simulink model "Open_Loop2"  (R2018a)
settings: Solver=VariableStepAuto  StartTime=0.0  StopTime=50  FixedStep=Ts  MaxStep=0.05  RelTol=1e-3  EnableMultiTasking=on
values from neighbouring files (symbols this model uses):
  Ax = 54.8    [init.m]
  Mlh2 = 41.12    [init.m]
  Mlox = 119.3    [init.m]
  Zeta = 0.002    [init.m]
undefined symbols (not defined in the file or in its folder): Aa, Av2, Ba, Bv2, Ca, Cv2, Da, Dv2, Kmix, Kq

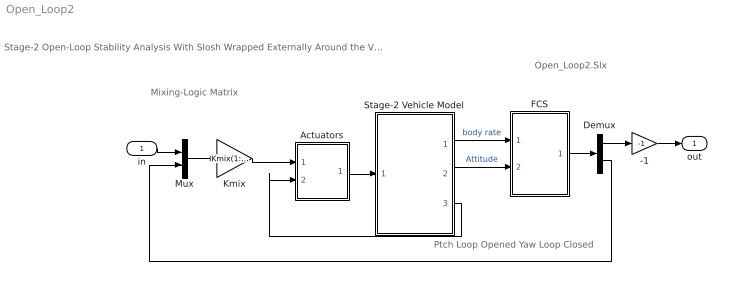
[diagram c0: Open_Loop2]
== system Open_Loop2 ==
  note: Stage-2 Open-Loop Stability Analysis With Slosh Wrapped Externally Around the Vehicle
  note: Mixing-Logic Matrix
  note: Ptch Loop Opened Yaw Loop Closed
  note: Open_Loop2.Slx
  in : Inport
  -1 : Gain  Gain=-1
  Actuators : Subsystem
  Demux : Demux  Outputs=2
  FCS : Subsystem
  Kmix : Gain  Gain=Kmix(1:2,2:3)  Multiplication=Matrix(K*u)
  Mux : Mux  Inputs=2
  Stage-2 Vehicle Model : Subsystem
  out : Outport
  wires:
  Stage-2 Vehicle Model/1(Wb) -> FCS/1(rate)  "body rate"
  Stage-2 Vehicle Model/2(atti) -> FCS/2(atter)  "Attitude"
  FCS/1(DQ,DR) -> Demux/1
  -1/1 -> out/1
  Actuators/1(del) -> Stage-2 Vehicle Model/1(dy,dz)
  Kmix/1 -> Actuators/1(dc)
  Mux/1 -> Kmix/1
  in/1 -> Mux/1
  Demux/1 -> -1/1
  Demux/2 -> Mux/2
  Stage-2 Vehicle Model/3(TL) -> Actuators/2(TL)

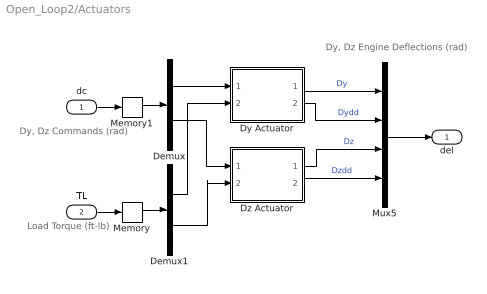
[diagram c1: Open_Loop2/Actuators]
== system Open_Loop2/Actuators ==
  note: Dy, Dz Engine Deflections (rad)
  note: Load Torque (ft-lb)
  note: Dy, Dz Commands (rad)
  dc : Inport
  TL : Inport  Port=2
  Demux : Demux  Outputs=2
  Demux1 : Demux  Outputs=2
  Dy Actuator : Subsystem
  Dz Actuator : Subsystem
  Memory : Memory
  Memory1 : Memory
  Mux5 : Mux
  del : Outport
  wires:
  Demux1/1 -> Dy Actuator/2(TL)
  Mux5/1 -> del/1
  Demux1/2 -> Dz Actuator/2(TL)
  Demux/2 -> Dz Actuator/1(dc)
  Dy Actuator/1(del) -> Mux5/1  "Dy"
  Dy Actuator/2(ddd) -> Mux5/2  "Dydd"
  Demux/1 -> Dy Actuator/1(dc)
  Dz Actuator/1(del) -> Mux5/3  "Dz"
  Dz Actuator/2(ddd) -> Mux5/4  "Dzdd"
  dc/1 -> Memory1/1
  TL/1 -> Memory/1
  Memory/1 -> Demux1/1
  Memory1/1 -> Demux/1

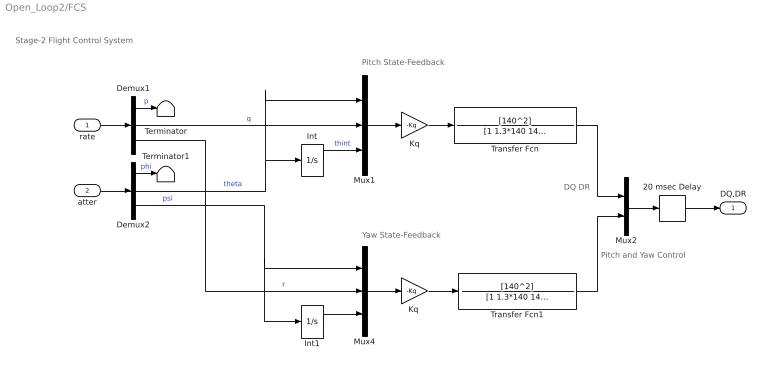
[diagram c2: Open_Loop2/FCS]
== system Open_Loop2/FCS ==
  note: Stage-2 Flight Control System
  note: Pitch and Yaw Control
  note: Yaw State-Feedback
  note: Pitch State-Feedback
  note: DQ DR
  rate : Inport
  atter : Inport  Port=2
  20 msec Delay : TransportDelay  DelayTime="[1  1]*0.020"  InitialOutput=[0 0]  PadeOrder=2
  Demux1 : Demux  Outputs=3
  Demux2 : Demux  Outputs=3
  Int : Integrator
  Int1 : Integrator
  Kq : Gain  Gain=-Kq  Multiplication=Matrix(K*u)
  "Kq " : Gain  Gain=-Kq  Multiplication=Matrix(K*u)
  Mux1 : Mux  Inputs=3
  Mux2 : Mux  Inputs=2
  Mux4 : Mux  Inputs=3
  Terminator : Terminator
  Terminator1 : Terminator
  Transfer Fcn : TransferFcn  Numerator=[140^2]  Denominator=[1 1.3*140 140^2]
  Transfer Fcn1 : TransferFcn  Numerator=[140^2]  Denominator=[1 1.3*140 140^2]
  DQ,DR : Outport
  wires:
  20 msec Delay/1 -> DQ,DR/1
  Demux2/1 -> Terminator1/1  "phi"
  Demux1/1 -> Terminator/1  "p"
  "Kq "/1 -> Transfer Fcn1/1
  Mux4/1 -> "Kq "/1
  Transfer Fcn1/1 -> Mux2/2
  Transfer Fcn/1 -> Mux2/1
  Mux1/1 -> Kq/1
  atter/1 -> Demux2/1
  Demux2/3 -> Mux4/1, Int1/1  "psi"
  Demux1/3 -> Mux4/2  "r"
  Int1/1 -> Mux4/3
  Int/1 -> Mux1/3  "thint"
  Demux1/2 -> Mux1/2  "q"
  Demux2/2 -> Int/1, Mux1/1  "theta"
  Kq/1 -> Transfer Fcn/1
  rate/1 -> Demux1/1
  Mux2/1 -> 20 msec Delay/1

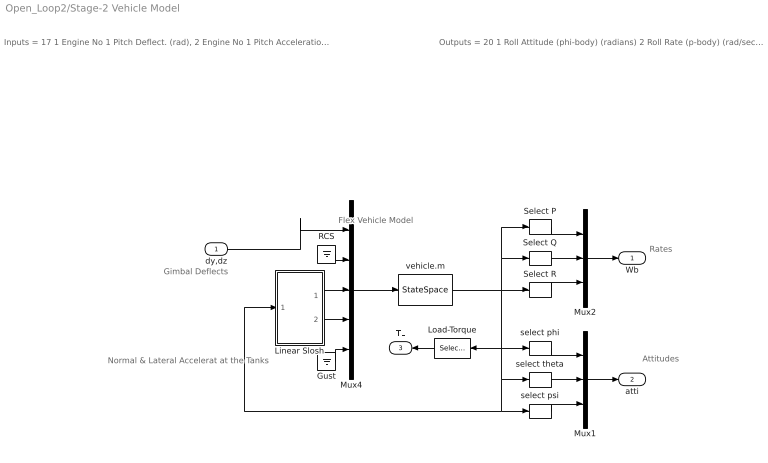
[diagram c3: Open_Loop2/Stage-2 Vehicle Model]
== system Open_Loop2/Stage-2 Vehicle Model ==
  note: Gimbal Deflects
  note: Flex Vehicle Model
  note: Outputs = 20 1 Roll Attitude (phi-body) (radians) 2 Roll Rate (p-body) (rad/sec) 3 Pitch Attitude (thet-bdy) (radians) 4 Pitch Rate (q-body) (rad/sec) 5 Yaw Attitude (psi-body) (radians) 6 Yaw Rate (r-body) (rad/sec) 7 Angle of attack, alfa, (radians) 8 Angle of sideslip, beta, (radian) 9 Change in Altitude, delta-h, (feet) 10 Forward Acceleration (V-dot) (ft/sec) 11 Cross Range Velocity (Vcr) (ft/sec) 12 Rate-Gyro # 1, Roll Rate (Body) (rad/sec) 13 Rate-Gyro # 2, Pitch Rate (Body) (rad/sec) 14 Rate-Gyro # 3, Yaw Rate (Body) (rad/sec) 15 Accelerat # 1, at LOX (along Y), (ft/sec^2) 16 Accelerat # 2, at LOX (along Z), (ft/sec^2) 17 Accelerat # 3, at LH2 (along Y), (ft/sec^2) 18 Accelerat # 4, at LH2 (along Z), (ft/sec^2) 19 Ptch Engine Load-Torque Tly (ft-lb) 20 Yaw Engine Load-Torque Tlz (ft-lb)
  note: Inputs = 17 1 Engine No 1 Pitch Deflect. (rad), 2 Engine No 1 Pitch Acceleration (rad/sec^2) 3 Engine No 1 Yaw Deflect. (rad), 4 Engine No 1 Yaw Acceleration (rad/sec^2) 5 RCS 1 Throttle Input dTh/Th 6 RCS 2 Throttle Input dTh/Th 7 RCS 3 Throttle Input dTh/Th 8 RCS 4 Throttle Input dTh/Th 9 LOX Force along Y-axis 10 LOX Force along Z-axis 11 LH2 Force along Y-axis 12 LH2 Force along Z-axis 13 Ext LOX Pitch Torque Inp 1 (ft-lb) 14 Ext LOX Yaw Torque Input 2 (ft-lb) 15 Ext LH2 Pitch Torque Inp 3 (ft-lb) 16 Ext LH2 Yaw Torque Input 4 (ft-lb) 17 Wind Gust Velocity (ft/sec)
  note: Attitudes
  note: Rates
  note: Normal & Lateral Accelerat at the Tanks
  dy,dz : Inport
  Gust : Ground
  Linear Slosh : Subsystem
  Load-Torque : Selector  InputPortWidth=20  IndexOptions=Index vector (dialog)  Indices=[19, 20]  OutputSizes=1
  Mux1 : Mux  Inputs=3
  Mux2 : Mux  Inputs=3
  Mux4 : Mux  Inputs=[4,4,4,4,1]
  RCS : Ground
  Select P : Selector  InputPortWidth=20  IndexOptions=Index vector (dialog)  Indices=[12]  OutputSizes=1
  Select Q : Selector  InputPortWidth=20  IndexOptions=Index vector (dialog)  Indices=[13]  OutputSizes=1
  Select R : Selector  InputPortWidth=20  IndexOptions=Index vector (dialog)  Indices=[14]  OutputSizes=1
  select phi : Selector  InputPortWidth=20  IndexOptions=Index vector (dialog)  Indices=[1]  OutputSizes=1
  select psi : Selector  InputPortWidth=20  IndexOptions=Index vector (dialog)  Indices=[5]  OutputSizes=1
  select theta : Selector  InputPortWidth=20  IndexOptions=Index vector (dialog)  Indices=[3]  OutputSizes=1
  vehicle.m : StateSpace  A=Av2  B=Bv2  C=Cv2  D=Dv2  InitialCondition=0
  Wb : Outport
  atti : Outport  Port=2
  TL : Outport  Port=3
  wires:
  Load-Torque/1 -> TL/1
  dy,dz/1 -> Mux4/1
  Select P/1 -> Mux2/1
  Select R/1 -> Mux2/3
  Mux1/1 -> atti/1
  select theta/1 -> Mux1/2
  Select Q/1 -> Mux2/2
  select phi/1 -> Mux1/1
  select psi/1 -> Mux1/3
  Mux2/1 -> Wb/1
  RCS/1 -> Mux4/2
  vehicle.m/1 -> Load-Torque/1, Linear Slosh/1(Ayz), select psi/1, select theta/1, select phi/1, Select R/1, Select P/1, Select Q/1
  Gust/1 -> Mux4/5
  Mux4/1 -> vehicle.m/1
  Linear Slosh/1(Fy,Fz) -> Mux4/3
  Linear Slosh/2(My,Mz) -> Mux4/4

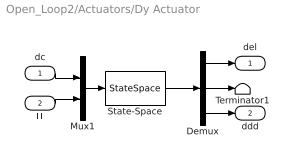
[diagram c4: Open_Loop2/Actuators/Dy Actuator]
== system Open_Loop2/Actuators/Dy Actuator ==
  dc : Inport
  TL : Inport  Port=2
  Demux : Demux  Outputs=3
  Mux1 : Mux  Inputs=2
  State-Space : StateSpace  A=Aa  B=Ba  C=Ca  D=Da  InitialCondition=0
  Terminator1 : Terminator
  del : Outport
  ddd : Outport  Port=2
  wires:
  Demux/1 -> del/1
  Demux/2 -> Terminator1/1
  Demux/3 -> ddd/1
  Mux1/1 -> State-Space/1
  State-Space/1 -> Demux/1
  dc/1 -> Mux1/1
  TL/1 -> Mux1/2

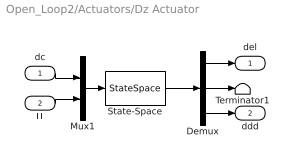
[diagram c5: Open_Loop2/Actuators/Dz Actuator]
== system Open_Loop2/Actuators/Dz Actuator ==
  dc : Inport
  TL : Inport  Port=2
  Demux : Demux  Outputs=3
  Mux1 : Mux  Inputs=2
  State-Space : StateSpace  A=Aa  B=Ba  C=Ca  D=Da  InitialCondition=0
  Terminator1 : Terminator
  del : Outport
  ddd : Outport  Port=2
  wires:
  Demux/1 -> del/1
  Demux/2 -> Terminator1/1
  Demux/3 -> ddd/1
  Mux1/1 -> State-Space/1
  State-Space/1 -> Demux/1
  dc/1 -> Mux1/1
  TL/1 -> Mux1/2

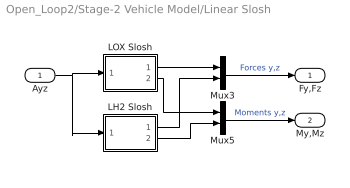
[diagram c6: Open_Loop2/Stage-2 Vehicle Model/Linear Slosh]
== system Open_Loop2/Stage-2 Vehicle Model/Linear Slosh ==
  Ayz : Inport
  LH2 Slosh : Subsystem
  LOX Slosh : Subsystem
  Mux3 : Mux  Inputs=[2, 2]
  Mux5 : Mux  Inputs=[2, 2]
  Fy,Fz : Outport
  My,Mz : Outport  Port=2
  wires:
  Ayz/1 -> LH2 Slosh/1(Ayz), LOX Slosh/1(Ayz)
  Mux3/1 -> Fy,Fz/1  "Forces y,z"
  LH2 Slosh/1(Fh2) -> Mux3/2
  LH2 Slosh/2(Mh2) -> Mux5/2
  LOX Slosh/1(Fox) -> Mux3/1
  Mux5/1 -> My,Mz/1  "Moments y,z"
  LOX Slosh/2(Mox) -> Mux5/1

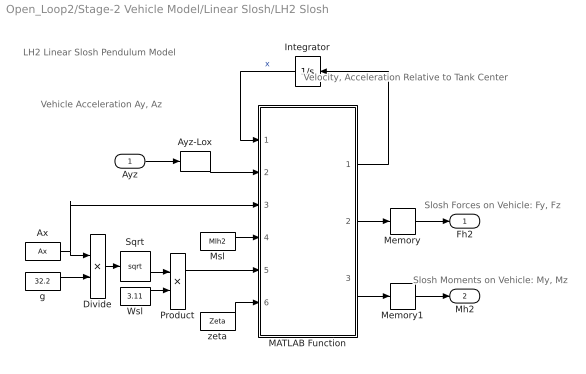
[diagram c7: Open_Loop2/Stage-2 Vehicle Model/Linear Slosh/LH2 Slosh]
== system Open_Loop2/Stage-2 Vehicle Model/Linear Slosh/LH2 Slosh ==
  note: LH2 Linear Slosh Pendulum Model
  note: Vehicle Acceleration Ay, Az
  note: Velocity, Acceleration Relative to Tank Center
  note: Slosh Forces on Vehicle: Fy, Fz
  note: Slosh Moments on Vehicle: My, Mz
  Ayz : Inport
  Ax : Constant  Value=Ax
  Ayz-Lox : Selector  InputPortWidth=20  IndexOptions=Index vector (dialog)  Indices=[17,18]  OutputSizes=1
  Divide : Product  Inputs=*/
  Integrator : Integrator
  MATLAB Function : MATLAB Function  TreatAsAtomicUnit=on
  Memory : Memory
  Memory1 : Memory
  Msl : Constant  Value=Mlh2
  Product : Product
  Sqrt : Sqrt
  Wsl : Constant  Value=3.11
  g : Constant  Value=32.2
  zeta : Constant  Value=Zeta
  Fh2 : Outport
  Mh2 : Outport  Port=2
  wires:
  MATLAB Function/2(F) -> Memory/1
  MATLAB Function/1(xd) -> Integrator/1
  Product/1 -> MATLAB Function/5(Ws)
  Wsl/1 -> Product/2
  Sqrt/1 -> Product/1
  Divide/1 -> Sqrt/1
  g/1 -> Divide/2
  Ax/1 -> MATLAB Function/3(Ax), Divide/1
  Integrator/1 -> MATLAB Function/1(x)  "x"
  Ayz/1 -> Ayz-Lox/1
  Memory/1 -> Fh2/1
  Ayz-Lox/1 -> MATLAB Function/2(Acc)
  Msl/1 -> MATLAB Function/4(Msl)
  zeta/1 -> MATLAB Function/6(zeta)
  Memory1/1 -> Mh2/1
  MATLAB Function/3(M) -> Memory1/1

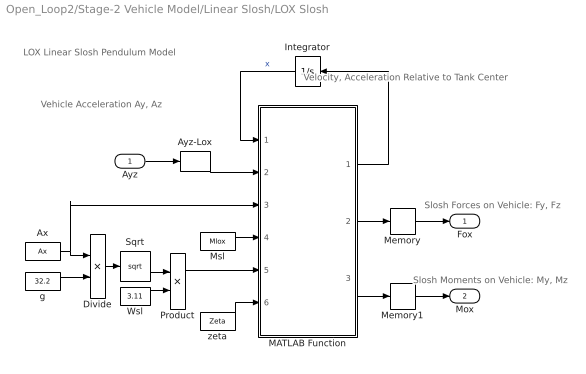
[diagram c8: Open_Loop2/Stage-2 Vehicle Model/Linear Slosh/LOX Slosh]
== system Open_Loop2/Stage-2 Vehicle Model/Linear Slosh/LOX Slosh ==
  note: LOX Linear Slosh Pendulum Model
  note: Vehicle Acceleration Ay, Az
  note: Velocity, Acceleration Relative to Tank Center
  note: Slosh Forces on Vehicle: Fy, Fz
  note: Slosh Moments on Vehicle: My, Mz
  Ayz : Inport
  Ax : Constant  Value=Ax
  Ayz-Lox : Selector  InputPortWidth=20  IndexOptions=Index vector (dialog)  Indices=[15,16]  OutputSizes=1
  Divide : Product  Inputs=*/
  Integrator : Integrator
  MATLAB Function : MATLAB Function  TreatAsAtomicUnit=on
  Memory : Memory
  Memory1 : Memory
  Msl : Constant  Value=Mlox
  Product : Product
  Sqrt : Sqrt
  Wsl : Constant  Value=3.11
  g : Constant  Value=32.2
  zeta : Constant  Value=Zeta
  Fox : Outport
  Mox : Outport  Port=2
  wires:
  MATLAB Function/2(F) -> Memory/1
  MATLAB Function/1(xd) -> Integrator/1
  Product/1 -> MATLAB Function/5(Ws)
  Wsl/1 -> Product/2
  Sqrt/1 -> Product/1
  Divide/1 -> Sqrt/1
  g/1 -> Divide/2
  Ax/1 -> MATLAB Function/3(Ax), Divide/1
  Integrator/1 -> MATLAB Function/1(x)  "x"
  Ayz/1 -> Ayz-Lox/1
  Memory/1 -> Fox/1
  Ayz-Lox/1 -> MATLAB Function/2(Acc)
  Msl/1 -> MATLAB Function/4(Msl)
  zeta/1 -> MATLAB Function/6(zeta)
  Memory1/1 -> Mox/1
  MATLAB Function/3(M) -> Memory1/1

== matlab function Open_Loop2/Stage-2
Vehicle Model/Linear 
Slosh/LH2 Slosh/MATLAB Function ==
function [xd,F,M] = Slosh_Lin(x,Acc,Ax, Msl,Ws,zeta) 
% Computes the slosh forces as a funct of 
% Acc(2)= Vehicle y,z Acceleration at Slosh
% x(l) = Ys_dot                             % Slosh Mass Veloc along Y 
% x(2) = Ys                                 % Slosh Mass Posit along Y 
% x(3) = Zs_dot                             % Slosh Mass Veloc along Z 
% x(4) = Zs                                 % Slosh Mass Posit along Z 
% F(1,2)= Fy, Fz                            % Forces Y,Z on the Vehicle
xd=zeros(4,1);
F=zeros(2,1); M=F;

% Slosh Mass Veloc & Accelerat along y and z 
xd(1)= -Ws^2*x(2) -Acc(1) -2*zeta*Ws*x(1);   % Ys_dd 
xd(2)=  x(1);                                % Ys_d 
xd(3)= -Ws^2*x(4) -Acc(2) -2*zeta*Ws*x(3);   % Zs_dd 
xd(4)=  x(3);                                % Zs_d 
F(1:2)= Msl*Ws^2*[x(2);x(4)] ...             % Fy,Fz Slosh Forces
       +Msl*2*zeta*Ws*[x(1);x(3)];
M(1:2)=-Msl*Ax*[x(4);-x(2)];                 % My,Mz Slosh Moments
end

== matlab function Open_Loop2/Stage-2
Vehicle Model/Linear 
Slosh/LOX Slosh/MATLAB Function ==
function [xd,F,M] = Slosh_Lin(x,Acc,Ax, Msl,Ws,zeta) 
% Computes the slosh forces as a funct of 
% Acc(2)= Vehicle y,z Acceleration at Slosh
% x(l) = Ys_dot                             % Slosh Mass Veloc along Y 
% x(2) = Ys                                 % Slosh Mass Posit along Y 
% x(3) = Zs_dot                             % Slosh Mass Veloc along Z 
% x(4) = Zs                                 % Slosh Mass Posit along Z 
% F(1,2)= Fy, Fz                            % Forces Y,Z on the Vehicle
xd=zeros(4,1);
F=zeros(2,1); M=F;

% Slosh Mass Veloc & Accelerat along y and z 
xd(1)= -Ws^2*x(2) -Acc(1) -2*zeta*Ws*x(1);   % Ys_dd 
xd(2)=  x(1);                                % Ys_d 
xd(3)= -Ws^2*x(4) -Acc(2) -2*zeta*Ws*x(3);   % Zs_dd 
xd(4)=  x(3);                                % Zs_d 
F(1:2)= Msl*Ws^2*[x(2);x(4)] ...             % Fy,Fz Slosh Forces
       +Msl*2*zeta*Ws*[x(1);x(3)];
M(1:2)=-Msl*Ax*[x(4);-x(2)];                 % My,Mz Slosh Moments
end
